FUNCTION_BLOCK FB_SignalHandlingDelayEdges EXTENDS FB_SignalHandlingDelay
VAR_OUTPUT
	bEdgeOn				: BOOL;
	bEdgeOff			: BOOL;
END_VAR
VAR
	fbRTriggerEdgeOn	: R_TRIG;
	fbFTriggerEdgeOff	: F_TRIG;
END_VAR

// =========================================================
;
// =========================================================

METHOD PUBLIC M_SetOutput
VAR_INPUT
END_VAR
// =========================================================
	// Calling method M_SetOutput of base class FB_InputSignalDelay via 'SUPER^.'
	
SUPER^.M_SetOutput();

// =========================================================
	// Edge on
	
rtrigEdgeOn(CLK := bInput);

bEdgeOn := rtrigEdgeOn.Q;

// =========================================================
	// Edge off
	
ftrigEdgeOff(CLK := bInput );	

bEdgeOff := ftrigEdgeOff.Q;

// =========================================================
END_METHOD

END_FUNCTION_BLOCK
